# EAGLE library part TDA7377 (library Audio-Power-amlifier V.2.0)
The TDA7377 is a new technology class AB car radio amplifier able to work either in DUAL BRIDGE or QUAD SINGLE ENDED configuration. The exclusive fully complementary structure of the output stage and the internally fixed gain guarantees the highest possible power performances with extremely reduced component count. The on-board clip detector simplifies gain compression operation. The fault diagnostics makes it possible to detect mistakes during car radio set assembly and wiring in the car
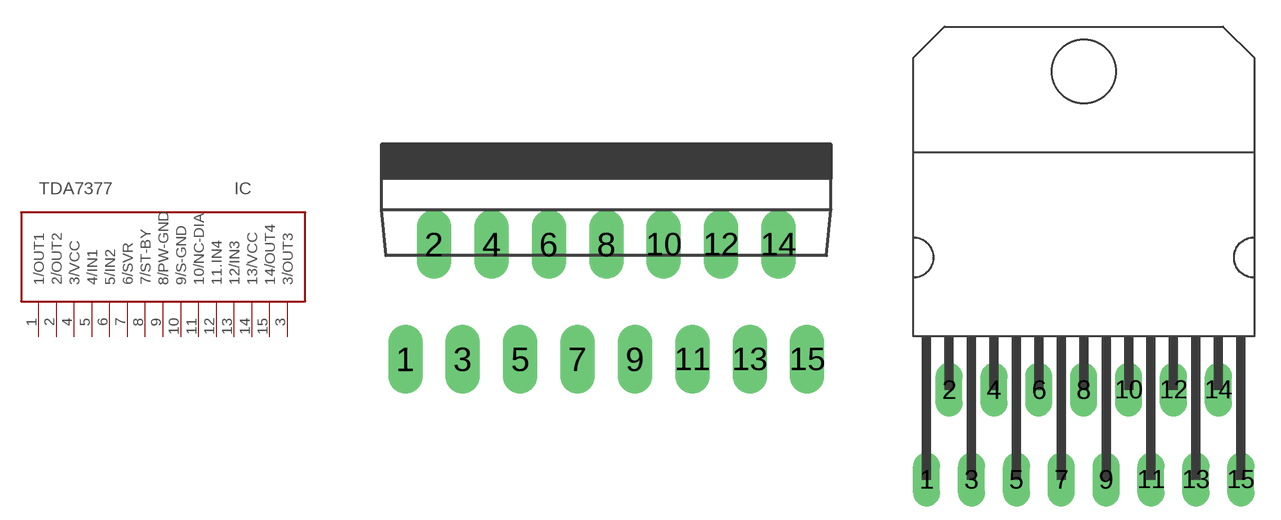
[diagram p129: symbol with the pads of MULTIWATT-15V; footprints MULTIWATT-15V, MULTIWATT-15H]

Designator prefix IC

## TDA7377TDA7377V  [MULTIWATT-15V]
1  1/OUT1  out
2  2/OUT2  out
3  3/OUT3  out
4  3/VCC  pwr
5  4/IN1  in
6  5/IN2  in
7  6/SVR
8  7/ST-BY
9  8/PW-GND  pwr
10  9/S-GND  pwr
11  10/NC-DIA  nc
12  11.IN4  in
13  12/IN3  in
14  13/VCC  pwr
15  14/OUT4  out

## TDA7377TDA7377H  [MULTIWATT-15H]
Pads as for MULTIWATT-15V

## Footprint MULTIWATT-15V (pad centres in mm)
Multiwatt 15 vertical
drill 1.016 long: 1 -8.89,-5.08; 2 -7.62,0; 3 -6.35,-5.08; 4 -5.08,0; 5 -3.81,-5.08; 6 -2.54,0; 7 -1.27,-5.08; 8 0,0; 9 1.27,-5.08; 10 2.54,0; 11 3.81,-5.08; 12 5.08,0; 13 6.35,-5.08; 14 7.62,0; 15 8.89,-5.08

## Footprint MULTIWATT-15H (pad centres in mm)
Multiwatt 15 horizontal
drill 1.016 long: 1 -8.89,-5.08; 2 -7.62,0; 3 -6.35,-5.08; 4 -5.08,0; 5 -3.81,-5.08; 6 -2.54,0; 7 -1.27,-5.08; 8 0,0; 9 1.27,-5.08; 10 2.54,0; 11 3.81,-5.08; 12 5.08,0; 13 6.35,-5.08; 14 7.62,0; 15 8.89,-5.08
